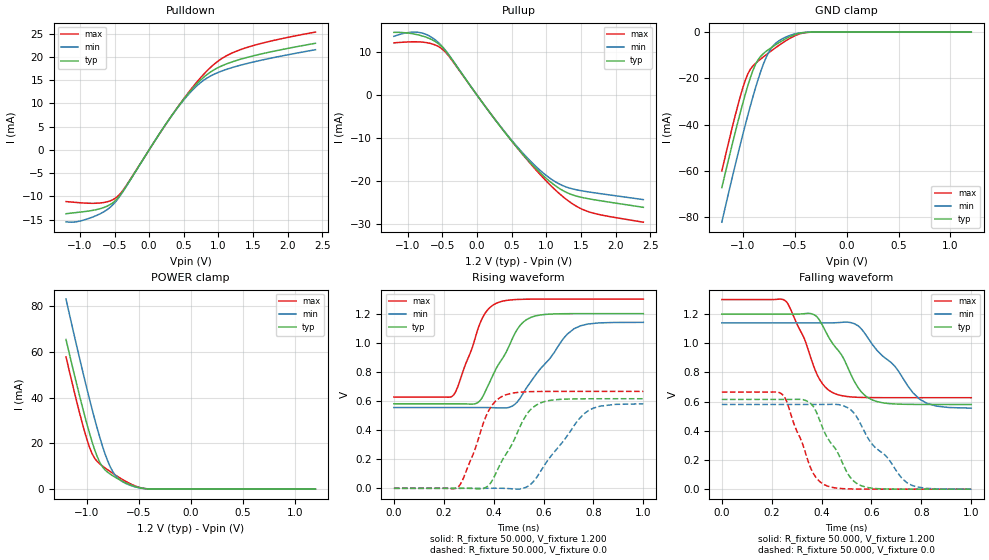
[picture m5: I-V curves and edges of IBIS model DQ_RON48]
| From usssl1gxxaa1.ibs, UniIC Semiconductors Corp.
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|   Model DQ_RON48
[Model] DQ_RON48
Model_type I/O
Vinl =  0.500V
Vinh =  0.700V
Vmeas =  0.600V
Rref =  50.000
Vref =  0.600V
C_comp   1.373pF   1.353pF   1.403pF
[Model Spec]
Vinh   0.700V   0.670V   0.750V
Vinl   0.500V   0.470V   0.550V
Vmeas   0.600V   0.570V   0.650V
Vref   0.600V   0.570V   0.650V
Rref   50.000   NA   NA
[Temperature Range]   25.000   0.125k   -40.000
[Voltage Range]   1.200V   1.140V   1.300V
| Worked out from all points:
|   slope of the pulldown table from 0 to 0.18 V, typ, clamps not added: 43.2 ohm
|   slope of the pullup table from 0 to 0.18 V, typ, clamps not added: 45.2 ohm
|   GND clamp passes 1 mA (typ) near -0.49 V on its own axis
|   POWER clamp passes 1 mA (typ) near -0.53 V on its own axis
|   rising waveform, R_fixture 50.000, V_fixture 1.200: 20-80 % time 112ps typ, 152ps min, 84.6ps max; typ from 0.581 V to 1.2 V
|   rising waveform, R_fixture 50.000, V_fixture 0.0: 20-80 % time 112ps typ, 148ps min, 86.6ps max; typ from 0 V to 0.615 V
|   falling waveform, R_fixture 50.000, V_fixture 1.200: 20-80 % time 126ps typ, 170ps min, 96.5ps max; typ from 1.2 V to 0.581 V
|   falling waveform, R_fixture 50.000, V_fixture 0.0: 20-80 % time 112ps typ, 152ps min, 86.1ps max; typ from 0.615 V to 0 V
[Pulldown]
|Voltage   I(typ)   I(min)   I(max)
-1.2V     -13.75mA   -15.49mA   -11.13mA
-1.015V   -13.43mA   -15.38mA   -11.37mA
-756mV    -12.85mA   -14.1mA    -11.48mA
-571mV    -11.85mA   -12.47mA   -11.03mA
-460mV    -10.51mA   -10.73mA   -10.1mA
-349mV    -8.251mA   -8.322mA   -8.093mA
354mV     7.964mA    7.903mA    7.965mA
613mV     12.96mA    12.66mA    13.2mA
798mV     15.75mA    15.08mA    16.42mA
1.02V     17.87mA    16.79mA    19.36mA
1.279V    19.31mA    18.05mA    21.34mA
2.4V      22.93mA    21.54mA    25.33mA
[Pullup]
|Voltage   I(typ)   I(min)   I(max)
-1.2V     14.6mA     13.68mA    12.16mA
-1.004V   14.45mA    14.54mA    12.37mA
-819mV    13.89mA    14.54mA    12.37mA
-634mV    12.76mA    13.22mA    11.85mA
-486mV    10.89mA    11.01mA    10.48mA
106mV     -2.363mA   -2.346mA   -2.332mA
513mV     -10.91mA   -10.74mA   -10.91mA
846mV     -17mA      -16.53mA   -17.31mA
1.142V    -21.2mA    -20.26mA   -22.23mA
1.364V    -23.11mA   -21.73mA   -25.12mA
1.586V    -24.02mA   -22.44mA   -26.97mA
2.4V      -26.08mA   -24.29mA   -29.54mA
[GND_clamp]
|Voltage   I(typ)   I(min)   I(max)
-1.2V     -67.26mA   -82.22mA   -60.1mA
-1.05V    -39.62mA   -53.62mA   -32.4mA
-1V       -31.05mA   -44.64mA   -24.37mA
-950mV    -23.16mA   -36.01mA   -18.1mA
-925mV    -19.62mA   -31.85mA   -16.02mA
-875mV    -13.89mA   -23.97mA   -13.48mA
-800mV    -9.288mA   -13.81mA   -10.72mA
-750mV    -7.535mA   -8.829mA   -8.993mA
-675mV    -5.274mA   -4.578mA   -6.506mA
-525mV    -1.587mA   -1.138mA   -2.208mA
-375mV    -90.13uA   -87.27uA   -132.9uA
1.2V      0A         0A         0A
[POWER_clamp]
|Voltage   I(typ)   I(min)   I(max)
-1.2V     65.51mA    83.21mA    57.91mA
-1.05V    37.38mA    53.57mA    29.99mA
-1V       28.74mA    44.18mA    21.95mA
-950mV    20.85mA    35.16mA    15.65mA
-925mV    17.34mA    30.84mA    13.56mA
-875mV    11.74mA    22.7mA     11.06mA
-800mV    7.436mA    12.47mA    8.502mA
-750mV    5.864mA    7.69mA     6.933mA
-675mV    3.901mA    3.837mA    4.735mA
-525mV    971.5uA    903.1uA    1.25mA
-400mV    85.95uA    125.9uA    91.19uA
1.2V      0A         0A         0A
[Ramp]
| variable   typ   min   max
dV/dt_r   0.369/0.112n   0.348/0.148n   0.400/86.560p
dV/dt_f   0.372/0.125n   0.351/0.170n   0.404/96.543p
R_load = 50.000
[Rising Waveform]
R_fixture= 50.000
V_fixture= 1.200
V_fixture_min= 1.140
V_fixture_max= 1.300
|time   V(typ)   V(min)   V(max)
0s        580.6mV    554.9mV    627mV
233ps     580.7mV    554.9mV    631.4mV
255ps     580.6mV    554.9mV    693.3mV
339ps     592.4mV    555.1mV    1.105V
376ps     700.4mV    554.6mV    1.226V
419ps     850.2mV    552.7mV    1.277V
486ps     1.067V     578.7mV    1.296V
556ps     1.178V     749.5mV    1.299V
722ps     1.2V       1.096V     1.3V
1ns       1.2V       1.14V      1.3V
[Rising Waveform]
R_fixture= 50.000
V_fixture= 0.0
V_fixture_min= 0.0
V_fixture_max= 0.0
|time   V(typ)   V(min)   V(max)
0s        42.45nV    734.6nV    24.88nV
259ps     100.6uV    -5.765uV   11.35mV
321ps     -1.418mV   -14.18uV   248.2mV
372ps     9.306mV    140.2uV    506.1mV
406ps     93.07mV    383.3uV    595.9mV
449ps     233.6mV    -765.1uV   642.3mV
531ps     505.1mV    8.021mV    662.9mV
590ps     588mV      121.8mV    665.3mV
781ps     615.1mV    535.3mV    665.9mV
1ns       615.4mV    580.4mV    665.9mV
[Falling Waveform]
R_fixture= 50.000
V_fixture= 1.200
V_fixture_min= 1.140
V_fixture_max= 1.300
|time   V(typ)   V(min)   V(max)
0s        1.2V       1.14V      1.3V
256ps     1.2V       1.14V      1.29V
330ps     1.203V     1.14V      1.035V
374ps     1.192V     1.14V      817.1mV
414ps     1.088V     1.14V      701.2mV
455ps     974.5mV    1.141V     653.8mV
546ps     697mV      1.121V     629.8mV
605ps     610.6mV    988.9mV    627.6mV
793ps     580.9mV    617.1mV    627mV
1ns       580.6mV    555.5mV    627mV
[Falling Waveform]
R_fixture= 50.000
V_fixture= 0.0
V_fixture_min= 0.0
V_fixture_max= 0.0
|time   V(typ)   V(min)   V(max)
0s        615.4mV    580.6mV    665.9mV
244ps     615.3mV    580.6mV    646.6mV
357ps     585.6mV    580.5mV    141.8mV
383ps     512.9mV    580.6mV    68.56mV
424ps     349.3mV    581.1mV    20.99mV
506ps     102.8mV    556.8mV    1.95mV
561ps     22.32mV    431.2mV    394.2uV
604ps     6.558mV    305.6mV    112.6uV
742ps     124.5uV    44.44mV    2.027uV
1ns       105.3nV    41.51uV    17.29nV
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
